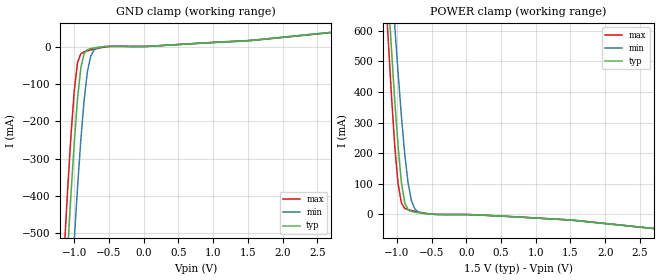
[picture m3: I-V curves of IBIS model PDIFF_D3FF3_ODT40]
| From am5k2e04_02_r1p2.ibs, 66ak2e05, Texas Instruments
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|   Model PDIFF_D3FF3_ODT40
[Model] PDIFF_D3FF3_ODT40
Model_type   Input
Polarity   Non-Inverting
Enable   Active-High
C_comp   3.323pF   3.247pF   3.424pF
C_comp_pullup   608.965fF   564.467fF   664.429fF
C_comp_pulldown 2.708pF   2.677pF   2.754pF
Vinh = 925.000mV
Vinl = 575.000mV
[Temperature Range]   25.000   125.000   -40.000
[Voltage Range]   1.500V   1.425V   1.575V
[GND Clamp Reference]   0.00V   0.00V   0.00V
|[C Comp Corner]
| variable   typ   min   max
|C_comp 3.323pF   3.424pF   3.247pF
|C_comp_pullup 608.965fF   664.429fF   564.467fF
|C_comp_pulldown 2.708pF   2.754pF   2.677pF
[POWER Clamp Reference]   1.500V   1.425V   1.575V
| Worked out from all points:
|   GND clamp passes 1 mA (typ) near -0.62 V on its own axis
|   POWER clamp passes 1 mA (typ) near -0.51 V on its own axis
[GND Clamp]
-1.48V    -1.899A    -2.158A    -1.745A
-1.145V   -711.1mA   -986.5mA   -544.5mA
-1.098V   -551.9mA   -826.5mA   -387.6mA
-1.05V    -400mA     -670.4mA   -242.3mA
-1.002V   -259.8mA   -520.2mA   -119.8mA
-954.6mV  -140.3mA   -378.8mA   -43.22mA
-906.8mV  -56.8mA    -250.5mA   -19.08mA
-859.1mV  -18.98mA   -143.1mA   -13.84mA
-811.4mV  -8.374mA   -66.55mA   -11.28mA
-763.6mV  -5.242mA   -25.26mA   -9.058mA
-668.2mV  -2.248mA   -3.26mA    -4.992mA
2.959V    43.1mA     43.04mA    42.16mA
[Power Clamp]
-1.459V   2.069A     2.186A     2.028A
-1.173V   901.2mA    1.117A     769.2mA
-1.125V   716.5mA    945.6mA    572.7mA
-1.077V   538.4mA    777.9mA    387.2mA
-1.03V    371mA      615.8mA    222.6mA
-981.8mV  221.5mA    461.7mA    99.84mA
-934.1mV  104.5mA    319.9mA    37.52mA
-886.4mV  38.14mA    197.3mA    19.98mA
-838.6mV  15.82mA    103.6mA    15.57mA
-790.9mV  9.974mA    45.65mA    12.95mA
-647.7mV  4.438mA    4.82mA     6.364mA
2.98V     -52.32mA   -52.48mA   -52.43mA
